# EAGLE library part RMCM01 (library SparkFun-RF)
Polar RMCM01 Heart Rate Monitor Receiver The Polar heart rate receiver component receiver wirelessly receives the heart rate signal from Polar transmitter belt. The complete heart rate measurement system consists of three different parts; transmitter, receiver and electronics and/or display device that is outputting the heart rate value. SparkFun Products Polar Heart Rate Monitor Interface (SEN-08661)
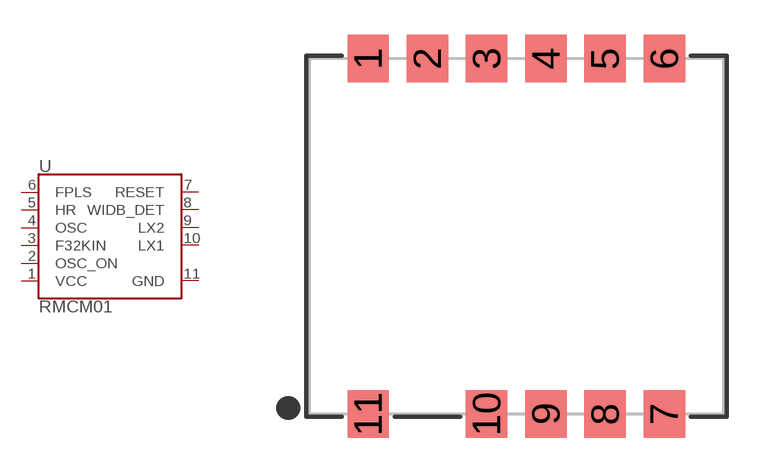
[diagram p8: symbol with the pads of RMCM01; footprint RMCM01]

Designator prefix -

## RMCM01 (PROD_ID: COMP-08853)  [RMCM01]
1  VCC
2  OSC_ON
3  F32KIN
4  OSC
5  HR
6  FPLS
7  RESET
8  WIDB_DET
9  LX2
10  LX1
11  GND

## Footprint RMCM01 (pad centres in mm)
Polar RMCM-01 Heart Rate Receiver Module Datasheet
smd 1.778 x 2.032: 1 -6.35,7.62; 2 -3.81,7.62; 3 -1.27,7.62; 4 1.27,7.62; 5 3.81,7.62; 6 6.35,7.62; 7 6.35,-7.62; 8 3.81,-7.62; 9 1.27,-7.62; 10 -1.27,-7.62; 11 -6.35,-7.62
